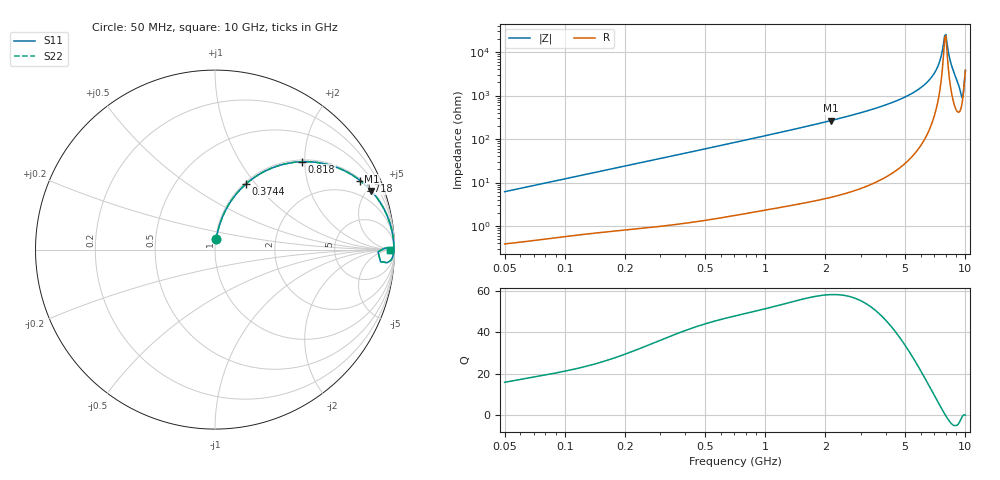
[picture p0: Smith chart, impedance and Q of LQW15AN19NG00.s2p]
!Murata Part Number: LQW15AN19NG00
!These Parameters are Measured in Series Mode Connection
!  o--[Z]--o
!Port1  Port2
!  o-------o
!Freq. Start=50[MHz] Stop=10[GHz], 401[Steps]
# Hz S RI R 50
!Freq.(Hz)	S 11(Real)	S 11(Imag)	S 21(Real)	S 21(Imag)	S 12(Real)	S 12(Imag)	S 22(Real)	S 22(Imag)
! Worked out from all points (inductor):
!   401 points, 50 MHz to 10 GHz, reference 50 ohm
!   read as one part in series: L = 19.5 nH near 51.34 MHz
!   highest Q = 58.2 at 2.123 GHz (marker M1), where L = 19.9 nH
!   self-resonance near 7.879 GHz
!   S11 on the Smith chart (normalised r, x): 50 MHz: 1.01, +0.12; 374.4 MHz: 1.02, +0.89; 818 MHz: 1.04, +1.94; 1.718 GHz: 1.07, +4.19; 10 GHz: 77, -2
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5e7  0.0076 0.0608  0.9924 -0.0608  0.9924 -0.0608  0.0076 0.0608
1.214486e8  0.027 0.1417  0.973 -0.1417  0.973 -0.1417  0.027 0.1417
2.949953e8  0.1165 0.3071  0.8835 -0.3071  0.8835 -0.3071  0.1165 0.3071
3.74422e8  0.1714 0.3645  0.8286 -0.3645  0.8286 -0.3645  0.1714 0.3645
7.071068e8  0.415 0.4824  0.585 -0.4824  0.585 -0.4824  0.415 0.4824
8.180189e8  0.486 0.4898  0.514 -0.4898  0.514 -0.4898  0.486 0.4898
1.717543e9  0.8104 0.3833  0.1896 -0.3833  0.1896 -0.3833  0.8104 0.3833
2.122994e9  0.8713 0.3264  0.1287 -0.3264  0.1287 -0.3264  0.8713 0.3264
4.171863e9  0.9739 0.1483  0.0261 -0.1483  0.0261 -0.1483  0.9739 0.1483
5.437278e9  0.9893 0.0868  0.0107 -0.0868  0.0107 -0.0868  0.9893 0.0868
6.54512e9  0.9948 0.0453  0.00516 -0.0453  0.00516 -0.0453  0.9948 0.0453
6.993273e9  0.9959 0.0303  0.0041 -0.0303  0.0041 -0.0303  0.9959 0.0303
7.276762e9  0.9963 0.0212  0.00372 -0.0212  0.00372 -0.0212  0.9963 0.0212
7.472112e9  0.9964 0.0149  0.00357 -0.0149  0.00357 -0.0149  0.9964 0.0149
7.775012e9  0.9964 0.00537  0.00356 -0.00537  0.00356 -0.00537  0.9964 0.00537
7.878683e9  0.9964 0.00208  0.00362 -0.00208  0.00362 -0.00208  0.9964 0.00208
7.983737e9  0.9963 -0.00127  0.00371 0.00127  0.00371 0.00127  0.9963 -0.00127
8.090191e9  0.9961 -0.0047  0.00385 0.0047  0.00385 0.0047  0.9961 -0.0047
8.530394e9  0.9949 -0.0196  0.00507 0.0196  0.00507 0.0196  0.9949 -0.0196
9.48396e9  0.9587 -0.0729  0.0413 0.0729  0.0413 0.0729  0.9587 -0.0729
9.610418e9  0.9222 -0.0674  0.0778 0.0674  0.0778 0.0674  0.9222 -0.0674
1e10  0.9745 -0.000728  0.0255 0.000728  0.0255 0.000728  0.9745 -0.000728
